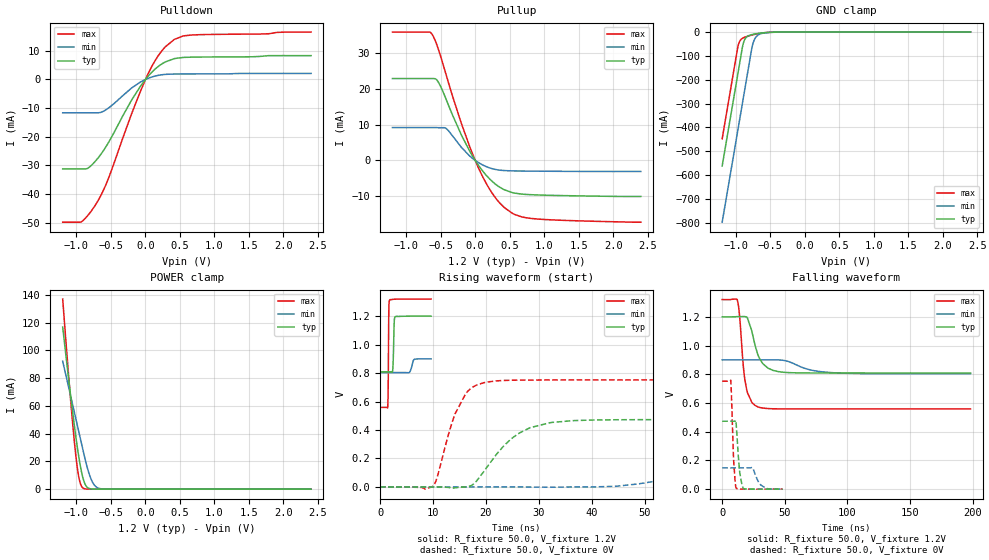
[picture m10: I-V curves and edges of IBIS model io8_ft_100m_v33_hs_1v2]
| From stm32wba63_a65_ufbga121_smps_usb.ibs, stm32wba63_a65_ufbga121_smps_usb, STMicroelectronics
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[Model]   io8_ft_100m_v33_hs_1v2
Model_type I/O
Polarity   Non-Inverting
Enable   Active-Low
| CAP_THRESHOLD on pad IOFT is "UDTCAPC" :
| Rising=30.0% of vddiom   Falling=70.0% of vddiom
| C_comp min and max val. don't necessarily correlate with the min and max pvt
| but are the smallest and greatest pad capacitance found.
| var   typ   min   max
C_comp   2.93789pF  2.85554pF  3.04885pF
|C_comp_pullup   1.70506pF  1.54588pF  1.84655pF
|C_comp_pulldown   1.23283pF  1.30965pF  1.20230pF
Vinl = 450.0mV
Vinh = 660.0mV
Vmeas = 600.0mV   | Reference voltage for timing measurements
Cref  = 50.0pF   | Timing specification test load capacitance value
Rref  = 1.0MOhm   | Timing specification test load resistance value
Vref  = 660.0mV   | Timing specification test load voltage
[Model Spec]
| TIME_THRESHOLD on pin ZIV33M is "CMOS" :
| Rising=50.0% of vddiom   Falling=50.0% of vddiom
Vinl 436.50000mV 331.50000mV 482.50000mV
Vinh 753.50000mV 549.50000mV 837.50000mV
| variable   typ   min   max
[Temperature Range] 25.0 140.0 -40.0
| variable   typ   min   max
[Voltage Range] 1.2V 900.0mV 1.32V
| variable   typ   min   max
[POWER Clamp Reference] 1.2V 900.0mV 1.32V
| variable   typ   min   max
[GND Clamp Reference] 0V 0V 0V
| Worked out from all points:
|   slope of the pulldown table from 0 to 0.18 V, typ, clamps not added: 40.6 ohm
|   slope of the pullup table from 0 to 0.18 V, typ, clamps not added: 39.4 ohm
|   GND clamp passes 1 mA (typ) near -0.51 V on its own axis
|   POWER clamp passes 1 mA (typ) near -0.83 V on its own axis
|   rising waveform, R_fixture 50.0, V_fixture 1.2V: 20-80 % time 157ps typ, 428ps min, 91.2ps max; typ from 0.809 V to 1.2 V
|   falling waveform, R_fixture 50.0, V_fixture 1.2V: 20-80 % time 8.58ns typ, 19.8ns min, 4.93ns max; typ from 1.2 V to 0.809 V
|   rising waveform, R_fixture 50.0, V_fixture 0V: 20-80 % time 6.99ns typ, 17.9ns min, 4.03ns max; typ from 0 V to 0.473 V
|   falling waveform, R_fixture 50.0, V_fixture 0V: 20-80 % time 2.69ns typ, 5.02ns min, 1.95ns max; typ from 0.473 V to 0 V
[POWER Clamp]
-1.2V     116.7mA    92.13mA    136.9mA
-1.09V    69.42mA    68.21mA    67.14mA
-1.02V    41.75mA    52.99mA    28.91mA
-990mV    30.98mA    46.47mA    16.09mA
-970mV    24.36mA    42.12mA    9.575mA
-940mV    15.59mA    35.6mA     3.485mA
-910mV    8.693mA    29.07mA    1.01mA
-860mV    2.259mA    18.59mA    104.6uA
-780mV    143.1uA    6.246mA    2.555uA
-720mV    16.22uA    1.846mA    157.1nA
-650mV    1.267uA    330.3uA    6.118nA
2.4V      0A         0A         0A
[GND Clamp]
-1.2V     -561.6mA   -797.4mA   -447.4mA
-980mV    -187.6mA   -423.4mA   -73.43mA
-960mV    -153.6mA   -389.4mA   -48.26mA
-900mV    -54.17mA   -287.4mA   -24.97mA
-870mV    -29.55mA   -236.4mA   -21.19mA
-830mV    -17.05mA   -168.4mA   -17.42mA
-760mV    -9.921mA   -54.55mA   -11.89mA
-730mV    -8.191mA   -29.78mA   -9.811mA
-690mV    -6.26mA    -14.49mA   -7.318mA
-600mV    -2.976mA   -4.315mA   -3.058mA
-380mV    -57.63uA   -251uA     -19.49uA
2.4V      872.7pA    204.8nA    349.4pA
| variable   typ   min   max
[Pullup Reference] 1.2V 900.0mV 1.32V
| variable   typ   min   max
[Pulldown Reference] 0V 0V 0V
[Pullup]
-1.2V     22.83mA    9.172mA    35.78mA
-660mV    22.82mA    9.172mA    35.78mA
-620mV    22.82mA    9.172mA    35.01mA
-540mV    21.98mA    9.134mA    31.33mA
-420mV    16.95mA    8.881mA    23.76mA
-200mV    7.069mA    3.642mA    10.26mA
0V        545.3fA    208.5pA    3fA
210mV     -5.173mA   -2.076mA   -8.052mA
420mV     -8.158mA   -2.82mA    -13.11mA
570mV     -9.105mA   -2.921mA   -15.05mA
790mV     -9.528mA   -2.972mA   -16.12mA
2.4V      -10.04mA   -3.075mA   -17.21mA
[Pulldown]
-1.2V     -31.2mA    -11.62mA   -49.78mA
-930mV    -31.2mA    -11.62mA   -49.64mA
-830mV    -30.86mA   -11.62mA   -47.25mA
-710mV    -28.04mA   -11.62mA   -43.19mA
-550mV    -22.55mA   -10.2mA    -35.3mA
-200mV    -7.146mA   -2.964mA   -11.89mA
40mV      1.171mA    405.8uA    2.092mA
130mV     3.416mA    1.118mA    6.182mA
230mV     5.302mA    1.613mA    9.763mA
420mV     7.288mA    1.898mA    13.99mA
670mV     7.779mA    1.924mA    15.51mA
2.4V      8.319mA    2.103mA    16.52mA
[Ramp]
dV/dt_r 283.79351mV/6.96724ns 88.92714mV/17.81644ns 450.99253mV/3.83261ns
dV/dt_f 234.6597mV/8.26019ns 57.89484mV/19.43934ns 456.73592mV/4.84752ns
R_load = 50.0
| Removed startup time: 0s 0s 0s  .
| Removed end time: 9.65ns.
[Rising Waveform]
R_fixture   = 50.0
V_fixture   = 1.2V
V_fixture_min = 900.0mV
V_fixture_max = 1.32V
0s        808.9mV    803.5mV    558.8mV
1.45ns    808.9mV    803.5mV    556.7mV
1.55ns    808.9mV    803.5mV    716.8mV
1.65ns    808.9mV    803.5mV    1.222V
1.8ns     808.9mV    803.5mV    1.312V
2.4ns     820.6mV    803.5mV    1.318V
2.5ns     897.1mV    803.5mV    1.318V
2.65ns    1.128V     803.5mV    1.319V
2.8ns     1.192V     803.5mV    1.319V
9.65ns    1.2V       899.5mV    1.32V
| Removed startup time: 0s 0s 0s  .
| Removed end time: 198.4ns.
[Falling Waveform]
R_fixture   = 50.0
V_fixture   = 1.2V
V_fixture_min = 900.0mV
V_fixture_max = 1.32V
0s        1.2V       900mV      1.32V
12.1ns    1.202V     900mV      1.318V
13.85ns   1.201V     900mV      1.211V
17.25ns   1.202V     900mV      824.1mV
19.6ns    1.199V     900mV      692mV
28.35ns   939.6mV    900.7mV    573.8mV
36.45ns   843.4mV    900.5mV    561.2mV
48.6ns    814.2mV    897.7mV    558.9mV
85.05ns   808.9mV    812.9mV    558.8mV
198.4ns   808.9mV    803.5mV    558.8mV
| Removed startup time: 0s 0s 0s  .
| Removed end time: 198.35ns.
[Rising Waveform]
R_fixture   = 50.0
V_fixture   = 0V
V_fixture_min = 0V
V_fixture_max = 0V
0s        4.83nV     215.5nV    3.39nV
9.95ns    -2.555uV   211.6nV    4.033mV
14ns      -7.431mV   171.4nV    494.9mV
16.2ns    -64.92uV   1.237uV    656.5mV
18.2ns    39.95mV    1.306uV    715.1mV
22.05ns   231.7mV    -661.6nV   745.2mV
28.35ns   416.2mV    -876.1uV   751.1mV
36.45ns   465.8mV    -142.8uV   751.5mV
81ns      472.9mV    140.4mV    751.6mV
198.3ns   473mV      148.2mV    751.7mV
| Removed startup time: 0s 0s 0s  .
| Removed end time: 48.4ns.
[Falling Waveform]
R_fixture   = 50.0
V_fixture   = 0V
V_fixture_min = 0V
V_fixture_max = 0V
0s        473mV      148.3mV    751.7mV
6.9ns     473mV      148.3mV    755.4mV
9.1ns     473mV      148.3mV    211.3mV
11.15ns   459.6mV    148.3mV    7.915mV
13.85ns   129.7mV    148.3mV    1.53mV
16.8ns    5.84mV     148.3mV    458.1uV
23.95ns   550uV      151.5mV    77.71uV
29.65ns   198.5uV    40.82mV    20.34uV
34.6ns    92.09uV    8.488mV    6.493uV
48.4ns    11.72uV    383.2uV    113.2nV
